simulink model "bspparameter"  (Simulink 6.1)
settings: Solver=VariableStepDiscrete  SolverMode=SingleTasking  StartTime=0.0  StopTime=500.0  FixedStep=0.01  RelTol=1e-3
PreLoadFcn:
  | bspparameter_ini
InitFcn:
  | bspparameter_ini
StopFcn:
  | bspparameter_plot
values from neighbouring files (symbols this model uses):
  Konst = 1.15    [bspparameter_ini.m]    (also in bsp_parameter_ini.m)
  verst = 10    [bspparameter_ini.m]    (also in bsp_parameter_ini.m)
libraries: simulink x1

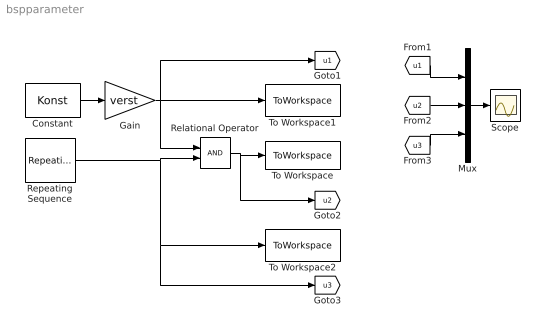
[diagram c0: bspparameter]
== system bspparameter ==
  Constant : Constant  Value=Konst
  Gain : Gain  Gain=verst
  Mux : Mux  Inputs=3
  Relational Operator : RelationalOperator
  Repeating Sequence : simulink/Sources/Repeating Sequence  rep_seq_t=zeit  rep_seq_y=wiederhol
  Scope : Scope
  To Workspace : ToWorkspace  VariableName=erg  SampleTime=-1  SaveFormat=Array
  To Workspace1 : ToWorkspace  VariableName=verst_Konst  SampleTime=-1  SaveFormat=Array
  To Workspace2 : ToWorkspace  VariableName=repeat  SampleTime=-1  SaveFormat=Array
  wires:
  Relational Operator/1 -> To Workspace/1, [u2]
  Constant/1 -> Gain/1
  Gain/1 -> Relational Operator/1, To Workspace1/1, [u1]
  Repeating Sequence/1 -> Relational Operator/2, To Workspace2/1, [u3]
  Mux/1 -> Scope/1
  [u1] -> Mux/1
  [u2] -> Mux/2
  [u3] -> Mux/3
